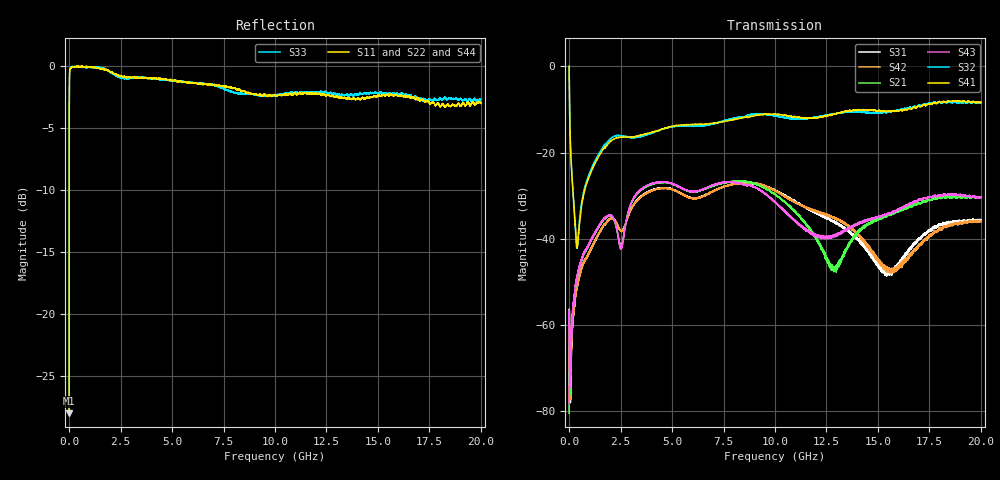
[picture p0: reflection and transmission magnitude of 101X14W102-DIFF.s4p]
!{101X14W102}
!Johanson Technology Inc.
!www.johansontechnology.com
!Test Board Conditions:
!Substrate Type  RO4350B
!Substrate Thickness  10 mil
!Substrate Dk  3.66
!TL Type: GCPW
!TL Trace Width  20 mil
!TL Gap  15 mil
!PART MODE DIFFERENTIAL
!DUT TOPOLOGY	DIFFERENTIAL 4-PORT
!Mounting Pad LxW  20x35 mil
# MHz S  dB  R 50
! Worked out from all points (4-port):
!   20001 points, 300 kHz to 20 GHz, reference 50 ohm
!   strongest paths, dB at 300 kHz, 5 GHz, 10 GHz, 15 GHz, 20 GHz:
!     S41: 0.0, -13.9, -11.1, -10.3, -8.4
!     S32: 0.0, -14.0, -11.5, -10.8, -8.4
!     S43: -78.2, -27.2, -31.5, -35.0, -30.3
!     S21: -80.4, -27.3, -29.7, -35.4, -30.3
!     S42: -70.3, -28.6, -28.8, -44.8, -35.9
!     S31: -76.1, -28.5, -28.7, -46.0, -35.7
!   lowest |S11| = -28.0 dB at 300 kHz (marker M1), VSWR 1.08, Z = 49.7 - j3.96 ohm
!   |S11| at or under -10 dB: start of sweep to 2.641 MHz
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0.3  -27.99 -92.2  -73.31 69.2  -75.38 114.0  -0.00 -2.4
     -80.44 100.8  -27.87 -95.4  -0.00 -2.3  -74.18 42.4
     -76.07 79.9  0.03 -2.2  -27.82 -94.8  -80.25 167.3
     -0.02 -2.5  -70.31 75.1  -78.19 117.2  -27.96 -90.4
395.294  -0.04 177.7  -48.79 83.0  -50.86 79.6  -42.23 2.2
         -48.71 80.0  -0.11 176.4  -41.65 13.8  -50.61 79.5
         -50.77 77.7  -41.67 12.5  -0.08 176.1  -48.60 79.7
         -42.12 2.5  -50.80 78.5  -48.53 79.8  -0.08 176.3
1628.276  -0.22 165.4  -35.79 50.6  -37.27 44.8  -19.40 63.4
          -35.81 51.1  -0.24 163.4  -18.83 61.1  -37.27 44.3
          -37.26 44.8  -18.83 61.1  -0.20 162.7  -35.69 50.1
          -19.40 63.2  -37.27 44.4  -35.70 49.9  -0.20 164.1
3838.242  -1.00 157.5  -27.66 66.3  -29.05 63.5  -15.51 32.8
          -27.71 66.2  -0.98 159.0  -15.78 30.8  -29.22 64.5
          -29.13 63.3  -15.77 30.7  -0.98 156.0  -27.53 64.9
          -15.54 32.7  -29.25 64.5  -27.53 64.8  -0.97 157.0
12875.11  -2.50 113.0  -46.78 -24.7  -36.01 -112.7  -11.02 -12.1
          -46.94 -24.4  -2.40 114.9  -10.96 -16.5  -34.90 -106.8
          -36.04 -113.0  -10.99 -16.3  -2.26 106.6  -39.18 -10.6
          -11.10 -12.1  -35.05 -107.2  -39.25 -11.0  -2.38 116.2
15483.07  -2.30 98.1  -34.52 12.8  -47.77 -75.9  -10.46 -24.7
          -34.53 13.0  -2.18 93.9  -10.68 -28.0  -47.30 -90.6
          -48.03 -76.2  -10.52 -28.9  -2.27 86.0  -34.15 -1.4
          -10.30 -24.2  -47.22 -92.8  -34.16 0.1  -2.29 88.6
20000  -3.02 72.1  -30.42 -28.0  -35.71 -76.1  -8.39 -45.7
       -30.32 -28.0  -3.15 69.5  -8.39 -51.2  -35.83 -73.3
       -35.73 -75.7  -8.38 -50.3  -2.73 58.0  -30.30 -39.6
       -8.40 -45.2  -35.94 -72.5  -30.35 -40.1  -2.89 64.7
